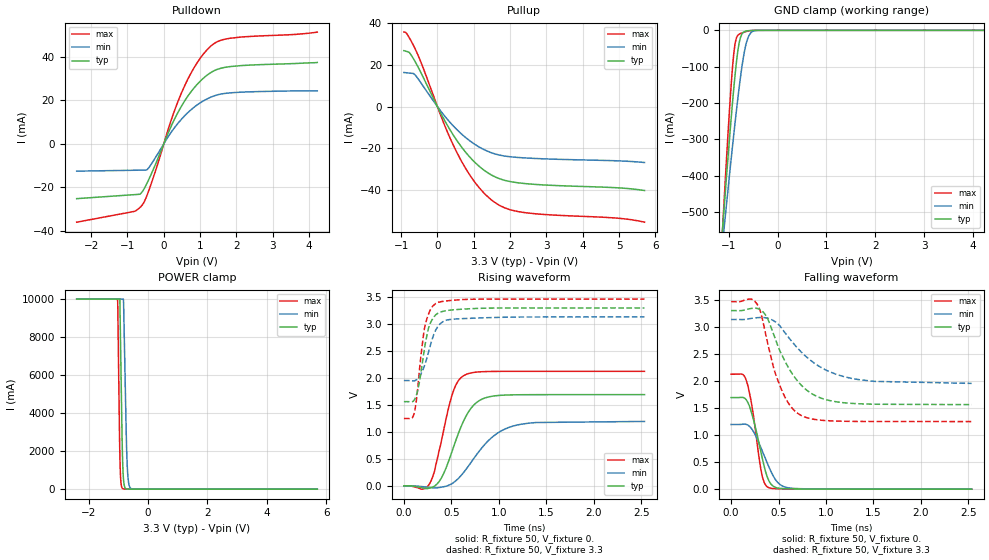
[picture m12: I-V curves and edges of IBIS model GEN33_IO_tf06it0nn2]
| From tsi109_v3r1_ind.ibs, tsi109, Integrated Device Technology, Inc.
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|   MODEL GEN33_IO_tf06it0nn2
[Model]   GEN33_IO_tf06it0nn2
Model_type  I/O
C_comp 1.25p 1.152p 1.348p
Polarity   Non-Inverting
Enable   Active-High
|   typ   min   max
Vinl   =   0.800v
Vinh   =   2.000v
Vmeas  =   1.65V
[Model Spec]
[Temperature Range]   25   125   -40
[Voltage Range] 3.3 3.135 3.465
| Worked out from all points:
|   slope of the pulldown table from 0 to 0.495 V, typ, clamps not added: 28.2 ohm
|   slope of the pullup table from 0 to 0.495 V, typ, clamps not added: 32.6 ohm
|   GND clamp passes 1 mA (typ) near -0.60 V on its own axis
|   POWER clamp passes 1 mA (typ) near -0.62 V on its own axis
|   rising waveform, R_fixture 50, V_fixture 0.: 20-80 % time 229ps typ, 344ps min, 168ps max; typ from 0 V to 1.69 V
|   rising waveform, R_fixture 50, V_fixture 3.3: 20-80 % time 103ps typ, 130ps min, 90ps max; typ from 1.56 V to 3.3 V
|   falling waveform, R_fixture 50, V_fixture 0.: 20-80 % time 136ps typ, 179ps min, 106ps max; typ from 1.69 V to 0 V
|   falling waveform, R_fixture 50, V_fixture 3.3: 20-80 % time 317ps typ, 447ps min, 225ps max; typ from 3.3 V to 1.56 V
[Pulldown]
-2.399V   -25.3mA    -12.63mA   -36.15mA
-811.5mV  -23.45mA   -12.21mA   -31.17mA
-603.9mV  -22.32mA   -12.16mA   -28.45mA
-416.4mV  -16.55mA   -11.09mA   -21.7mA
-175.3mV  -7.333mA   -4.867mA   -9.724mA
193mV     7.745mA    5.056mA    10.41mA
514.4mV   18.13mA    11.85mA    24.53mA
722mV     23.36mA    15.27mA    31.74mA
943mV     27.83mA    18.2mA     37.97mA
1.351V    33.37mA    21.85mA    45.79mA
1.82V     35.56mA    23.46mA    48.62mA
4.224V    37.46mA    24.37mA    51.46mA
[Pullup]
-924.3mV  26.91mA    16.42mA    35.82mA
-776.9mV  26mA       16.15mA    33.14mA
-622.9mV  21.88mA    15.39mA    28.08mA
-428.7mV  15.4mA     10.78mA    20.19mA
180.7mV   -6.081mA   -4.115mA   -8.231mA
528.9mV   -16.09mA   -10.9mA    -21.78mA
957.4mV   -25.45mA   -17.23mA   -34.52mA
1.466V    -32.59mA   -21.98mA   -44.46mA
1.855V    -35.36mA   -23.7mA    -48.58mA
2.424V    -36.91mA   -24.6mA    -50.88mA
4.888V    -38.85mA   -25.93mA   -53.4mA
5.699V    -40.21mA   -26.77mA   -55.42mA
[GND Clamp]
-2.399V   -2.991A    -2.405A    -3.89A
-1.155V   -594mA     -623.2mA   -610.1mA
-1.107V   -507.6mA   -558.2mA   -493.5mA
-1.083V   -465mA     -526mA     -436.3mA
-979.4mV  -286.4mA   -388.9mA   -203.9mA
-907.7mV  -173mA     -297.5mA   -76.38mA
-859.8mV  -106.6mA   -239mA     -28.75mA
-788.1mV  -34.55mA   -157mA     -10.67mA
-732.3mV  -10.47mA   -100.8mA   -7.132mA
-644.6mV  -2.072mA   -36.37mA   -3.26mA
-477.1mV  -97.48uA   -1.256mA   -161.8uA
4.224V    0A         0A         0A
[Power Clamp]
-2.399V   10A        10A        10A
-1.025V   10A        10A        10A
-1.018V   10A        10A        9.844A
-946.5mV  10A        10A        1.861A
-914.9mV  6.959A     10A        462.1mA
-851.8mV  1.453A     10A        28.06mA
-820.3mV  468mA      9.817A     10.6mA
-733.4mV  19.1mA     3.131A     4.039mA
-701.9mV  6.728mA    1.404A     3.278mA
-654.5mV  2.014mA    379.7mA    2.302mA
-583.5mV  582.8uA    49.6mA     1.138mA
5.699V    0A         0A         0A
[Ramp]
dV/dt_r 1.015/228.756p .717/344.077p 1.275/168.406p
dV/dt_f 1.043/317.591p .709/447.763p 1.33/225.281p
[Rising Waveform]
R_fixture = 50
V_fixture = 0.
0s        714nV      0V         582.7nV
270ps     -41.37mV   -28.72mV   36.89mV
325ps     -582.9uV   -39.73mV   288.4mV
390ps     132mV      -26.27mV   790.9mV
505ps     628mV      40.6mV     1.671V
565ps     928.7mV    122.6mV    1.927V
645ps     1.261V     284.1mV    2.059V
815ps     1.601V     691.3mV    2.116V
1.155ns   1.688V     1.111V     2.124V
2.535ns   1.692V     1.195V     2.125V
[Rising Waveform]
R_fixture = 50
V_fixture = 3.3
V_fixture_min = 3.135
V_fixture_max = 3.465
0s        1.562V     1.954V     1.249V
110ps     1.596V     1.949V     1.355V
135ps     1.703V     1.97V      1.627V
165ps     1.94V      2.03V      2.169V
215ps     2.523V     2.219V     2.907V
270ps     2.981V     2.548V     3.235V
345ps     3.186V     2.92V      3.393V
435ps     3.247V     3.066V     3.428V
575ps     3.272V     3.099V     3.45V
2.535ns   3.3V       3.135V     3.465V
[Falling Waveform]
R_fixture = 50
V_fixture = 0.
0s        1.692V     1.195V     2.125V
120ps     1.695V     1.199V     2.122V
165ps     1.636V     1.194V     1.983V
215ps     1.411V     1.118V     1.585V
315ps     678.9mV    762.5mV    350.5mV
350ps     411.9mV    613.4mV    119.8mV
395ps     167.6mV    425.2mV    29.01mV
490ps     21.57mV    126mV      8.027mV
630ps     6.368mV    18.7mV     3.312mV
2.535ns   12.24uV    11.96uV    22.03uV
[Falling Waveform]
R_fixture = 50
V_fixture = 3.3
V_fixture_min = 3.135
V_fixture_max = 3.465
0s        3.3V       3.135V     3.465V
275ps     3.339V     3.169V     3.415V
315ps     3.306V     3.172V     3.247V
380ps     3.168V     3.161V     2.738V
520ps     2.532V     3.002V     1.887V
630ps     2.171V     2.75V      1.524V
750ps     1.903V     2.515V     1.352V
960ps     1.675V     2.237V     1.272V
1.27ns    1.585V     2.047V     1.253V
2.535ns   1.562V     1.955V     1.249V
